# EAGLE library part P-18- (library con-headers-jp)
HEADER PLUG PINS
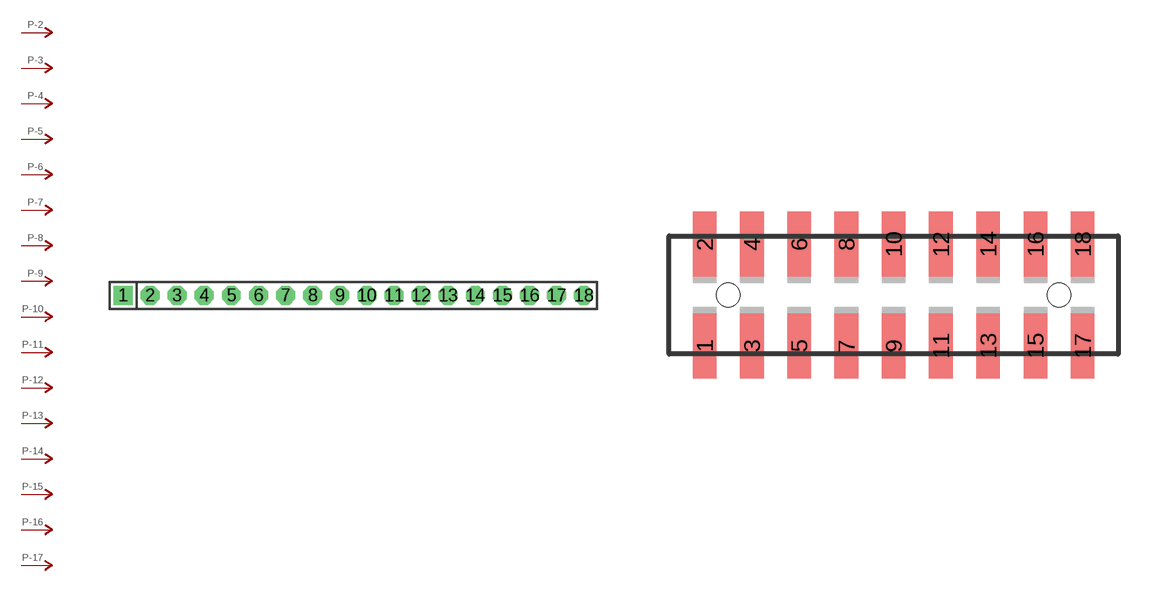
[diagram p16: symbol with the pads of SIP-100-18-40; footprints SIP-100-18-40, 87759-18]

Designator prefix P; gates -2=P-N -3=P-N -4=P-N -5=P-N -6=P-N -7=P-N -8=P-N -9=P-N -10=P-N -11=P-N -12=P-N -13=P-N -14=P-N -15=P-N -16=P-N -17=P-N -18=P-N -1=P-NV

## P-18-SIP-100-40  [SIP-100-18-40]
1  -1:P  pas
2  -2:P  pas
3  -3:P  pas
4  -4:P  pas
5  -5:P  pas
6  -6:P  pas
7  -7:P  pas
8  -8:P  pas
9  -9:P  pas
10  -10:P  pas
11  -11:P  pas
12  -12:P  pas
13  -13:P  pas
14  -14:P  pas
15  -15:P  pas
16  -16:P  pas
17  -17:P  pas
18  -18:P  pas

## P-18-87759  [87759-18]
Pads as for SIP-100-18-40

## P-18-100-2X09  [DIL-100-2X09]
Pads as for SIP-100-18-40

## P-18-100-2X09_M  [DIL-100-2X09_M]
Pads as for SIP-100-18-40

## P-18-2MM-2X09  [DIL-2MM-2X09]
Pads as for SIP-100-18-40

## P-18-2MM-2X09_M  [DIL-2MM-2X09_M]
Pads as for SIP-100-18-40

## P-18-SIP-100-32  [SIP-100-18-32]
Pads as for SIP-100-18-40

## P-18-SIP-100-40Y  [SIP-100-18-40Y]
Pads as for SIP-100-18-40

## P-18-SIP-100-32Y  [SIP-100-18-32Y]
Pads as for SIP-100-18-40

## P-18-87759_M  [87759-18_M]
Pads as for SIP-100-18-40

## Footprint SIP-100-18-40 (pad centres in mm)
SIP Header - 0.1", 40 mil drill
drill 1.016 pad 1.778 square: 1 -21.59,0
drill 1.016 pad 1.778 octagon: 2 -19.05,0; 3 -16.51,0; 4 -13.97,0; 5 -11.43,0; 6 -8.89,0; 7 -6.35,0; 8 -3.81,0; 9 -1.27,0; 10 1.27,0; 11 3.81,0; 12 6.35,0; 13 8.89,0; 14 11.43,0; 15 13.97,0; 16 16.51,0; 17 19.05,0; 18 21.59,0

## Footprint 87759-18 (pad centres in mm)
Molex PCB Pin Headers 2.00mm (.079") Pitch Milli-Grid Header, Vertical SMD
smd 1 x 2.75: 1 -8,-2.15; 2 -8,2.15; 3 -6,-2.15; 4 -6,2.15; 5 -4,-2.15; 6 -4,2.15; 7 -2,-2.15; 8 -2,2.15; 9 0,-2.15; 10 0,2.15; 11 2,-2.15; 12 2,2.15; 13 4,-2.15; 14 4,2.15; 15 6,-2.15; 16 6,2.15; 17 8,-2.15; 18 8,2.15
hole 1 at -7,0
hole 1 at 7,0

## Footprint DIL-100-2X09 (pad centres in mm)
PIN HEADER - 0.1"
drill 1.016 square: 1 -10.16,-1.27
drill 1.016 octagon: 2 -10.16,1.27; 3 -7.62,-1.27; 4 -7.62,1.27; 5 -5.08,-1.27; 6 -5.08,1.27; 7 -2.54,-1.27; 8 -2.54,1.27; 9 0,-1.27; 10 0,1.27; 11 2.54,-1.27; 12 2.54,1.27; 13 5.08,-1.27; 14 5.08,1.27; 15 7.62,-1.27; 16 7.62,1.27; 17 10.16,-1.27; 18 10.16,1.27

## Footprint DIL-100-2X09_M (pad centres in mm)
PIN HEADER - MIRRORED 0.1"
drill 1.016 square: 1 -10.16,1.27
drill 1.016 octagon: 2 -10.16,-1.27; 3 -7.62,1.27; 4 -7.62,-1.27; 5 -5.08,1.27; 6 -5.08,-1.27; 7 -2.54,1.27; 8 -2.54,-1.27; 9 0,1.27; 10 0,-1.27; 11 2.54,1.27; 12 2.54,-1.27; 13 5.08,1.27; 14 5.08,-1.27; 15 7.62,1.27; 16 7.62,-1.27; 17 10.16,1.27; 18 10.16,-1.27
